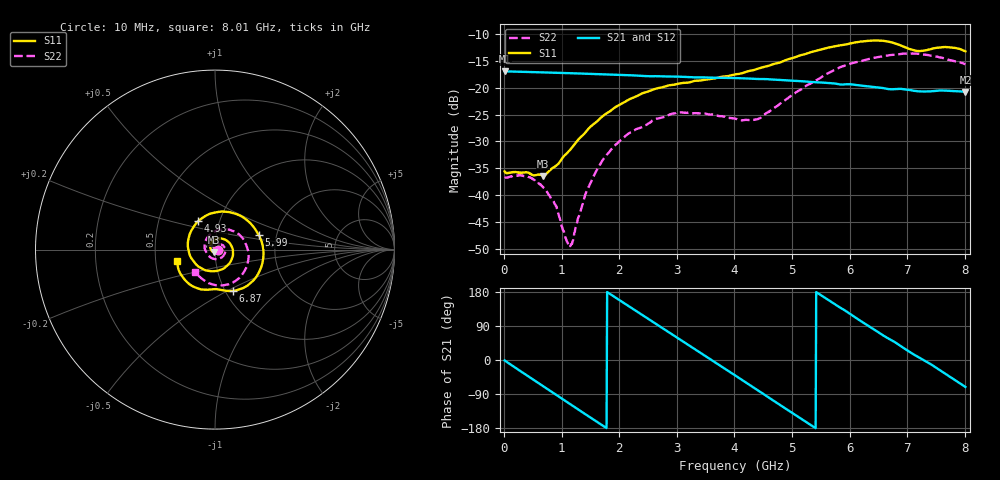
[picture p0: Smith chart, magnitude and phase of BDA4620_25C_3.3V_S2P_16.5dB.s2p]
!Agilent Technologies,E5071B,MY42404982,A.09.10
!Date: Wed May 06 08:52:09 2026
!Data & Calibration Information:
!Freq	S11:SOLT2(ON)	S21:SOLT2(ON)	S12:SOLT2(ON)	S22:SOLT2(ON)
# Hz S RI R 50
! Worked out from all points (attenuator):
!   801 points, 10 MHz to 8.01 GHz, reference 50 ohm
!   highest |S21| = -16.92 dB at 10 MHz (marker M1); lowest = -20.8 dB at 8.01 GHz (marker M2)
!   lowest |S11| = -36.4 dB at 680 MHz (marker M3), VSWR 1.03, Z = 49.6 - j1.44 ohm
!   |S11| at or under -10 dB: start of sweep to end of sweep
!   |S22| runs from -49.5 to -13.6 dB; largest |S21 - S12| = 0.00061
!   S11 on the Smith chart (normalised r, x): 10 MHz: 1.03, -0.00; 4.93 GHz: 0.79, +0.26; 5.99 GHz: 1.62, +0.28; 6.87 GHz: 1.08, -0.53; 8.01 GHz: 0.65, -0.08
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1e7  0.0166 -0.00118  0.1425 -0.00305  0.1427 -0.00306  0.0145 -0.000562
4.2e8  0.00862 -0.0137  0.1025 -0.0958  0.1026 -0.0961  0.0137 -0.00564
6.8e8  -0.0042 -0.0145  0.0491 -0.1303  0.049 -0.1305  0.00885 -0.00785
8.9e8  -0.0161 -0.00912  -0.00132 -0.138  -0.00153 -0.1384  0.00318 -0.00751
1.13e9  -0.0251 0.00643  -0.0573 -0.1243  -0.0575 -0.1246  -0.0027 -0.00212
1.19e9  -0.0259 0.0115  -0.0699 -0.1173  -0.0701 -0.1175  -0.00372 -9.15e-05
1.35e9  -0.025 0.0253  -0.099 -0.0928  -0.0991 -0.0929  -0.00547 0.0055
1.58e9  -0.0141 0.0448  -0.1261 -0.0464  -0.1262 -0.0465  -0.00443 0.0153
1.88e9  0.016 0.0608  -0.1308 0.0223  -0.1309 0.0223  0.00466 0.0269
2.68e9  0.0995 -0.00166  -0.00286 0.128  -0.0028 0.1282  0.0483 0.0191
3.4e9  0.0333 -0.1118  0.1174 0.0433  0.1175 0.0433  0.0452 -0.0361
4.01e9  -0.1009 -0.087  0.0937 -0.0799  0.0938 -0.0802  -0.015 -0.0494
4.42e9  -0.1508 0.0138  0.0183 -0.1195  0.0183 -0.1196  -0.0503 -0.012
4.93e9  -0.0947 0.1582  -0.0789 -0.0866  -0.079 -0.0868  -0.0414 0.0685
5.35e9  0.0427 0.2123  -0.1126 -0.0119  -0.1127 -0.0119  0.0248 0.1088
5.99e9  0.2441 0.0804  -0.0594 0.0902  -0.0596 0.0904  0.1532 0.0646
6.34e9  0.2646 -0.0722  0.0026 0.1028  0.00277 0.103  0.1851 -0.0123
6.68e9  0.1754 -0.204  0.0542 0.0806  0.0544 0.0808  0.1743 -0.0988
6.87e9  0.0978 -0.23  0.0765 0.0611  0.0766 0.0611  0.1497 -0.1421
7.19e9  0.00672 -0.22  0.0917 0.013  0.092 0.0131  0.0753 -0.1935
7.55e9  -0.1009 -0.2143  0.0856 -0.0396  0.0858 -0.0395  -0.0199 -0.1916
8.01e9  -0.2096 -0.0618  0.0297 -0.0865  0.0298 -0.0866  -0.1105 -0.1233
